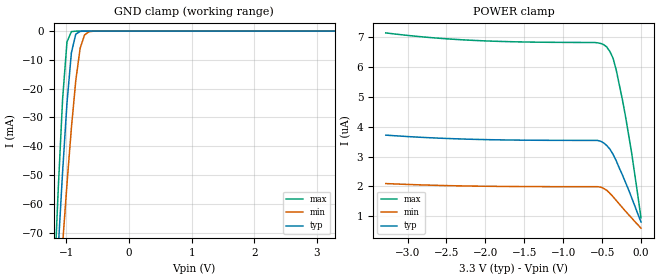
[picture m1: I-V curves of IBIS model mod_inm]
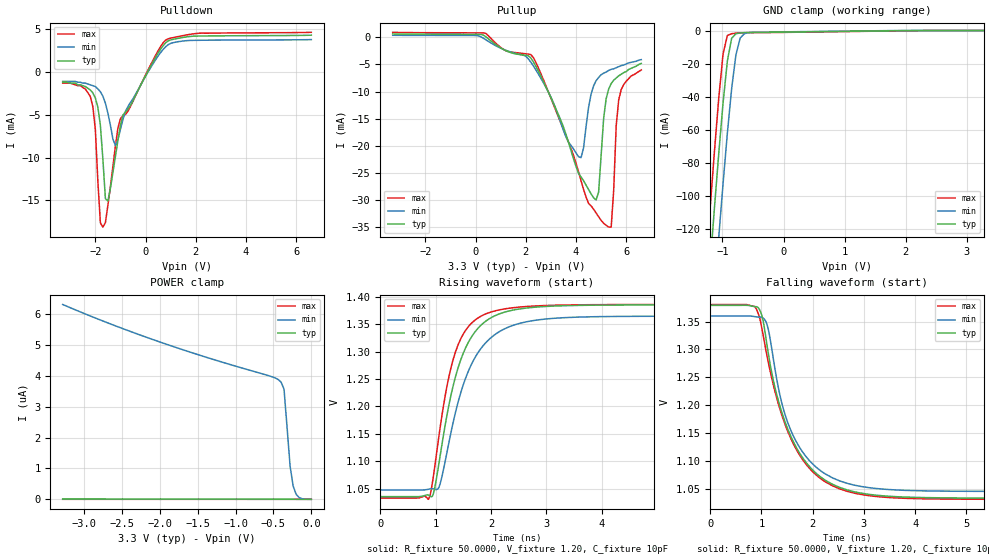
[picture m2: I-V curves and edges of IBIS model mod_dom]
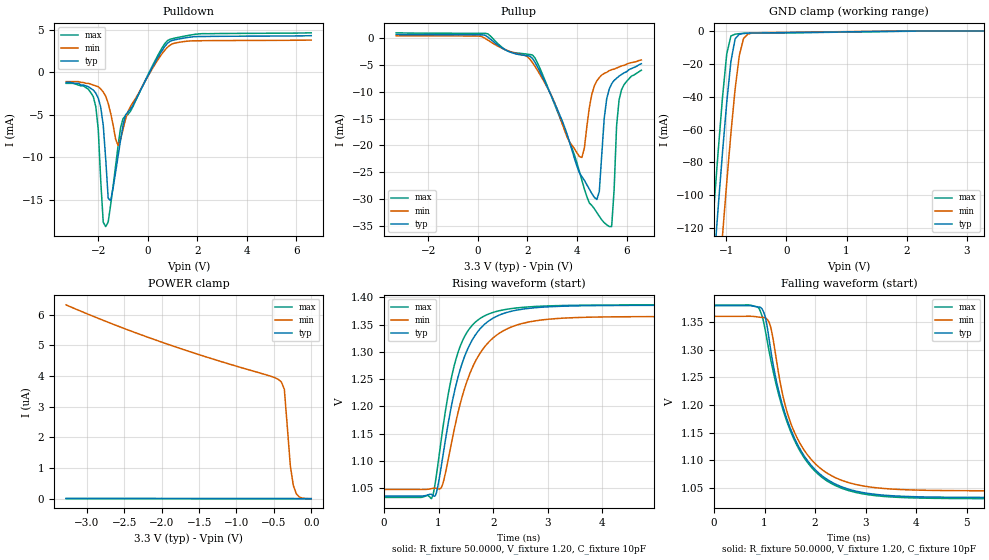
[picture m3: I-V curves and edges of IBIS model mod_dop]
| IBIS (I/O, Buffer, Information, Specification) Model, officially
| electronic behavioral standard for Buffer structures of digital pins.
[IBIS ver]  4.0
[File name] rhflvdsr2d2_3v3_rev3.ibs
[File Rev]  1.0
[Date]   26 May 2017
[Source]   CAD & Design Services (Catania) - STMicroelectronics
[Notes]
   (Note1)  This IBIS model is the model of the product with package
   (Flat18 package elements);
   (Note2)  This IBIS model is extracted with nominal 3.3V power supply
   (min:3.0V, typ:3.3V, max:3.6V)
   (Note3)  This IBIS model has some Notes about the non-monotonicity
   of the I-V curves, but they are not indicative of problems
   inside the model;
[Disclaimer] Customers are solely responsible for all aspects of their
   own product designs or applications using this IBIS Model.
   STMicroelectronics assumes no liability for Custmer
   Designs and applications associated to this IBIS Model.
   In the use of this IBIS Model Customer shall not modify,
   disassemble, alter this Model in whole or in part.
   If Customers do not accept these terms, the IBIS Model
   may not be used. For any problems or modifications please
   contact STMicroelectronics (www.st.com).
[Copyright] (c) 2017 STMicroelectronics
|   Component RHFLVDSR2D2
[Component] RHFLVDSR2D2
[Manufacturer] STMicroelectronics
[Package]
| variable   typ   min   max
R_pkg   0.0   0.0   0.0
L_pkg   0.0H   0.0H   0.0H
C_pkg   0.0F   0.0F   0.0F
[Pin]  signal_name   model_name   R_pin   L_pin   C_pin
1   RIN1M   mod_inm   0.0   0.0   0.0
2   RIN1P   mod_inp   0.0   0.0   0.0
3   RIN2P   mod_inp   0.0   0.0   0.0
4   RIN2M   mod_inm   0.0   0.0   0.0
5   REN2   mod_en   0.0   0.0   0.0
6   DO2M   mod_dom   0.0   0.0   0.0
7   DO2P   mod_dop   0.0   0.0   0.0
8   DO1P   mod_dop   0.0   0.0   0.0
9   DO1M   mod_dom   0.0   0.0   0.0
10   DEN1   mod_den   0.0   0.0   0.0
11   DIN1   mod_din   0.0   0.0   0.0
12   DIN2   mod_din   0.0   0.0   0.0
13   DEN2   mod_den   0.0   0.0   0.0
14   VCC   POWER   0.0   0.0   0.0
15   GND   GND   0.0   0.0   0.0
16   RO2   mod_out   0.0   0.0   0.0
17   RO1   mod_out   0.0   0.0   0.0
18   REN1   mod_en   0.0   0.0   0.0
[Diff pin]  inv_pin   vdiff   tdelay_typ  tdelay_min  tdelay_max
2   1   100mV   0.0s   0.0s   0.0s
3   4   100mV   0.0s   0.0s   0.0s
7   6   0.0   0.0s   0.0s   0.0s
8   9   0.0   0.0s   0.0s   0.0s
[Package Model]  313197_RHFLVDSR2D2_1
[Define Package Model]  313197_RHFLVDSR2D2_1
[Manufacturer]  STMicroelectronics
[OEM]  STMicroelectronics
[Description]  ceramic flat-18
[Number Of Pins]  18
[Pin Numbers]
|Pin Num   Terminal Name
1   |  NET1
2   |  NET2
3   |  NET3
4   |  NET4
5   |  NET5
6   |  NET6
7   |  NET7
8   |  NET8
9   |  NET9
10   |  NET10
11   |  NET11
12   |  NET12
13   |  NET13
14   |  NET14
15   |  NET15
16   |  NET16
17   |  NET17
18   |  NET18
[Model Data]
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[End Model Data]
[End Package Model]
| Models and submodels in the file (8): mod_inm (Input), mod_inp (Input), mod_dom (3-state), mod_dop (3-state), mod_den (Input), mod_din (Input), mod_out (3-state), mod_en (Input)
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|   Model mod_inm
[Model]   mod_inm
Model_type Input
Vinl   =   0.8000V
Vinh   =   2.0000V
C_comp   1.160pF   1.148pF   1.230pF
[Temperature Range]  25.0000   0.1250k   -55.0000
[Voltage Range]   3.3000V   3.0000V   3.6000V
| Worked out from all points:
|   GND clamp passes 1 mA (typ) near -0.85 V on its own axis
[GND_clamp]
|Voltage   I(typ)   I(min)   I(max)
-3.3V     -1.037A    -847.3mA   -1.291A
-1.2V     -103.9mA   -118.4mA   -90.61mA
-1.13V    -75.7mA    -95.97mA   -55.15mA
-1.06V    -48.92mA   -74.09mA   -23.64mA
-990mV    -24.98mA   -53.14mA   -3.768mA
-920mV    -7.585mA   -33.75mA   -179.6uA
-850mV    -1.057mA   -17.22mA   -5.053uA
-780mV    -97.1uA    -5.969mA   -122.7nA
-710mV    -6.82uA    -1.339mA   -2.974nA
-640mV    -449.9nA   -233.7uA   -80.51pA
-500mV    -1.943nA   -4.459uA   -7.043pA
3.28V     3.538uA    1.987uA    6.819uA
[POWER_clamp]
|Voltage   I(typ)   I(min)   I(max)
-3.28V    3.717uA    2.092uA    7.145uA
-2.24V    3.582uA    2.011uA    6.906uA
-560mV    3.539uA    1.988uA    6.813uA
-480mV    3.455uA    1.928uA    6.753uA
-440mV    3.369uA    1.867uA    6.673uA
-400mV    3.249uA    1.766uA    6.522uA
-360mV    3.079uA    1.654uA    6.302uA
-320mV    2.869uA    1.533uA    5.922uA
-240mV    2.389uA    1.289uA    4.922uA
-200mV    2.138uA    1.169uA    4.362uA
-120mV    1.618uA    937nA      3.121uA
0V        803nA      596.8nA    940.7nA
|   Model mod_dom
[Model]   mod_dom
Model_type 3-state
|Vinl   =   0.925V
|Vinh   =   1.650V
Polarity   Inverting
Enable   Active-Low
Vmeas  =   1.650V
Cref   =   10pF
C_comp   0.321pF   0.255pF   0.355pF
[Temperature Range]   25.0000   0.1250k   -55.0000
[Voltage Range]   3.3000V   3.0000V   3.6000V
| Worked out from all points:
|   slope of the pulldown table from 0 to 0.495 V, typ, clamps not added: 189 ohm
|   slope of the pullup table from 0 to 0.495 V, typ, clamps not added: 636 ohm
|   GND clamp passes 1 mA (typ) near -0.04 V on its own axis
|   rising waveform, R_fixture 50.0000, V_fixture 1.20, C_fixture 10pF: 20-80 % time 508ps typ, 593ps min, 416ps max; typ from 1.03 V to 1.39 V
|   falling waveform, R_fixture 50.0000, V_fixture 1.20, C_fixture 10pF: 20-80 % time 725ps typ, 659ps min, 752ps max; typ from 1.38 V to 1.03 V
[Pulldown]
|Voltage   I(typ)   I(min)   I(max)
-3.3V     -1.2mA     -1.1mA     -1.3mA
-2.2V     -2.1mA     -1.5mA     -2.87mA
-2V       -3.04mA    -1.7mA     -6.72mA
-1.9V     -4.11mA    -1.97mA    -12.77mA
-1.8V     -6.22mA    -2.31mA    -17.61mA
-1.7V     -10.17mA   -2.82mA    -18.12mA
-1.6V     -14.79mA   -3.64mA    -17.59mA
-1.5V     -15.07mA   -4.82mA    -15.56mA
-1.2V     -9.84mA    -8.59mA    -8.63mA
-900mV    -5.024mA   -5.524mA   -5.101mA
800mV     3.413mA    2.947mA    3.726mA
6.6V      4.296mA    3.783mA    4.632mA
[Pullup]
|Voltage   I(typ)   I(min)   I(max)
-3.3V     647.6uA    399.4uA    947.4uA
100mV     579.3uA    314.7uA    847.9uA
2.2V      -3.796mA   -4.572mA   -3.171mA
4.2V      -25.81mA   -22.22mA   -26.5mA
4.8V      -30.05mA   -8mA       -32.46mA
4.9V      -28.59mA   -7.39mA    -33.16mA
5.1V      -14.94mA   -6.6mA     -34.36mA
5.3V      -9.54mA    -6.1mA     -35.06mA
5.4V      -8.53mA    -5.9mA     -35.08mA
5.6V      -7.5mA     -5.6mA     -16.31mA
5.7V      -7.1mA     -5.4mA     -11.52mA
6.6V      -4.8mA     -4.1mA     -6mA
[GND_clamp]
|Voltage   I(typ)   I(min)   I(max)
-3.3V     -1.345A    -1.575A    -1.253A
-1.27V    -175.3mA   -229.2mA   -141.4mA
-1.2V     -140.6mA   -192.8mA   -106.4mA
-1.13V    -106.6mA   -158.1mA   -72.36mA
-1.06V    -73.96mA   -124.6mA   -40.43mA
-990mV    -43.62mA   -92.45mA   -14.06mA
-920mV    -18.43mA   -62.15mA   -2.993mA
-850mV    -4.705mA   -35.21mA   -1.919mA
-780mV    -1.922mA   -14.74mA   -1.598mA
-710mV    -1.49mA    -4.531mA   -1.403mA
-640mV    -1.316mA   -1.864mA   -1.318mA
3.28V     23.54pA    1.078uA    19.83pA
[POWER_clamp]
|Voltage   I(typ)   I(min)   I(max)
-3.28V    10.31nA    6.317uA    198.2pA
-2.68V    8.946nA    5.716uA    177.1pA
-2.04V    7.686nA    5.138uA    154.7pA
-560mV    5.402nA    4.006uA    102.7pA
-440mV    5.247nA    3.889uA    98.42pA
-400mV    5.194nA    3.807uA    96.77pA
-360mV    5.137nA    3.571uA    94.08pA
-280mV    4.92nA     1.078uA    85.8pA
-240mV    4.209nA    433.6nA    68.63pA
-200mV    1.594nA    161nA      33.42pA
-160mV    407.8pA    56.33nA    25.64pA
0V        24.13pA    1.061nA    22.9pA
[Ramp]
| variable   typ   min   max
dV/dt_r   0.4405/0.4439n   0.3885/0.4693n   0.4915/0.4754n
dV/dt_f   0.4405/0.2435n   0.3885/0.2716n   0.4915/0.2233n
R_load = 50.0000
[Rising Waveform]
R_fixture= 50.0000   |   New Rising 10pF
V_fixture= 1.20
V_fixture_min= 1.20
V_fixture_max= 1.20
C_fixture = 10pF
|time   V(typ)   V(min)   V(max)
0s        1.035V     1.047V     1.033V
870ps     1.038V     1.049V     1.03V
940ps     1.036V     1.05V      1.059V
1.08ns    1.109V     1.058V     1.16V
1.22ns    1.192V     1.124V     1.245V
1.36ns    1.255V     1.19V      1.3V
1.64ns    1.326V     1.275V     1.351V
1.98ns    1.361V     1.324V     1.372V
3.38ns    1.384V     1.362V     1.385V
10ns      1.385V     1.365V     1.386V
[Falling Waveform]
R_fixture= 50.0000   |  New Falling 10pF
V_fixture= 1.20
V_fixture_min= 1.20
V_fixture_max= 1.20
C_fixture = 10pF
|time   V(typ)   V(min)   V(max)
0s        1.379V     1.36V      1.381V
860ps     1.377V     1.359V     1.378V
1.05ns    1.342V     1.355V     1.317V
1.13ns    1.295V     1.337V     1.278V
1.29ns    1.222V     1.251V     1.215V
1.61ns    1.137V     1.147V     1.133V
1.99ns    1.084V     1.095V     1.081V
2.53ns    1.052V     1.064V     1.049V
3.93ns    1.034V     1.046V     1.032V
10ns      1.033V     1.045V     1.031V
|   Model mod_dop
[Model]   mod_dop
Model_type 3-state
|Vinl   =   0.925V
|Vinh   =   1.650V
Polarity   Non-Inverting
Enable   Active-High
Vmeas  =   1.650V
Cref   =   10pF
C_comp   0.321pF   0.255pF   0.355pF
[Temperature Range]   25.0000   0.1250k   -55.0000
[Voltage Range]   3.3000V   3.0000V   3.6000V
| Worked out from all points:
|   slope of the pulldown table from 0 to 0.495 V, typ, clamps not added: 189 ohm
|   slope of the pullup table from 0 to 0.495 V, typ, clamps not added: 636 ohm
|   GND clamp passes 1 mA (typ) near -0.04 V on its own axis
|   rising waveform, R_fixture 50.0000, V_fixture 1.20, C_fixture 10pF: 20-80 % time 508ps typ, 593ps min, 416ps max; typ from 1.03 V to 1.39 V
|   falling waveform, R_fixture 50.0000, V_fixture 1.20, C_fixture 10pF: 20-80 % time 725ps typ, 659ps min, 752ps max; typ from 1.38 V to 1.03 V
[Pulldown]
|Voltage   I(typ)   I(min)   I(max)
-3.3V     -1.2mA     -1.1mA     -1.3mA
-2.2V     -2.1mA     -1.5mA     -2.87mA
-2V       -3.04mA    -1.7mA     -6.72mA
-1.9V     -4.11mA    -1.97mA    -12.77mA
-1.8V     -6.22mA    -2.31mA    -17.61mA
-1.7V     -10.17mA   -2.82mA    -18.12mA
-1.6V     -14.79mA   -3.64mA    -17.59mA
-1.5V     -15.07mA   -4.82mA    -15.56mA
-1.2V     -9.84mA    -8.59mA    -8.63mA
-900mV    -5.024mA   -5.524mA   -5.101mA
800mV     3.413mA    2.947mA    3.726mA
6.6V      4.296mA    3.783mA    4.632mA
[Pullup]
|Voltage   I(typ)   I(min)   I(max)
-3.3V     647.6uA    399.4uA    947.4uA
100mV     579.3uA    314.7uA    847.9uA
2.2V      -3.796mA   -4.572mA   -3.171mA
4.2V      -25.81mA   -22.22mA   -26.5mA
4.8V      -30.05mA   -8mA       -32.46mA
4.9V      -28.59mA   -7.39mA    -33.16mA
5.1V      -14.94mA   -6.6mA     -34.36mA
5.3V      -9.54mA    -6.1mA     -35.06mA
5.4V      -8.53mA    -5.9mA     -35.08mA
5.6V      -7.5mA     -5.6mA     -16.31mA
5.7V      -7.1mA     -5.4mA     -11.52mA
6.6V      -4.8mA     -4.1mA     -6mA
[GND_clamp]
|Voltage   I(typ)   I(min)   I(max)
-3.3V     -1.345A    -1.575A    -1.253A
-1.27V    -175.3mA   -229.2mA   -141.4mA
-1.2V     -140.6mA   -192.8mA   -106.4mA
-1.13V    -106.6mA   -158.1mA   -72.36mA
-1.06V    -73.96mA   -124.6mA   -40.43mA
-990mV    -43.62mA   -92.45mA   -14.06mA
-920mV    -18.43mA   -62.15mA   -2.993mA
-850mV    -4.705mA   -35.21mA   -1.919mA
-780mV    -1.922mA   -14.74mA   -1.598mA
-710mV    -1.49mA    -4.531mA   -1.403mA
-640mV    -1.316mA   -1.864mA   -1.318mA
3.28V     23.54pA    1.078uA    19.83pA
[POWER_clamp]
|Voltage   I(typ)   I(min)   I(max)
-3.28V    10.31nA    6.317uA    198.2pA
-2.68V    8.946nA    5.716uA    177.1pA
-2.04V    7.686nA    5.138uA    154.7pA
-560mV    5.402nA    4.006uA    102.7pA
-440mV    5.247nA    3.889uA    98.42pA
-400mV    5.194nA    3.807uA    96.77pA
-360mV    5.137nA    3.571uA    94.08pA
-280mV    4.92nA     1.078uA    85.8pA
-240mV    4.209nA    433.6nA    68.63pA
-200mV    1.594nA    161nA      33.42pA
-160mV    407.8pA    56.33nA    25.64pA
0V        24.13pA    1.061nA    22.9pA
[Ramp]
| variable   typ   min   max
dV/dt_r   0.4405/0.4439n   0.3885/0.4693n   0.4915/0.4754n
dV/dt_f   0.4405/0.2435n   0.3885/0.2716n   0.4915/0.2233n
R_load = 50.0000
[Rising Waveform]
R_fixture= 50.0000   |   New Rising 10pF
V_fixture= 1.20
V_fixture_min= 1.20
V_fixture_max= 1.20
C_fixture = 10pF
|time   V(typ)   V(min)   V(max)
0s        1.035V     1.047V     1.033V
870ps     1.038V     1.049V     1.03V
940ps     1.036V     1.05V      1.059V
1.08ns    1.109V     1.058V     1.16V
1.22ns    1.192V     1.124V     1.245V
1.36ns    1.255V     1.19V      1.3V
1.64ns    1.326V     1.275V     1.351V
1.98ns    1.361V     1.324V     1.372V
3.38ns    1.384V     1.362V     1.385V
10ns      1.385V     1.365V     1.386V
[Falling Waveform]
R_fixture= 50.0000   |  New Falling 10pF
V_fixture= 1.20
V_fixture_min= 1.20
V_fixture_max= 1.20
C_fixture = 10pF
|time   V(typ)   V(min)   V(max)
0s        1.379V     1.36V      1.381V
860ps     1.377V     1.359V     1.378V
1.05ns    1.342V     1.355V     1.317V
1.13ns    1.295V     1.337V     1.278V
1.29ns    1.222V     1.251V     1.215V
1.61ns    1.137V     1.147V     1.133V
1.99ns    1.084V     1.095V     1.081V
2.53ns    1.052V     1.064V     1.049V
3.93ns    1.034V     1.046V     1.032V
10ns      1.033V     1.045V     1.031V
